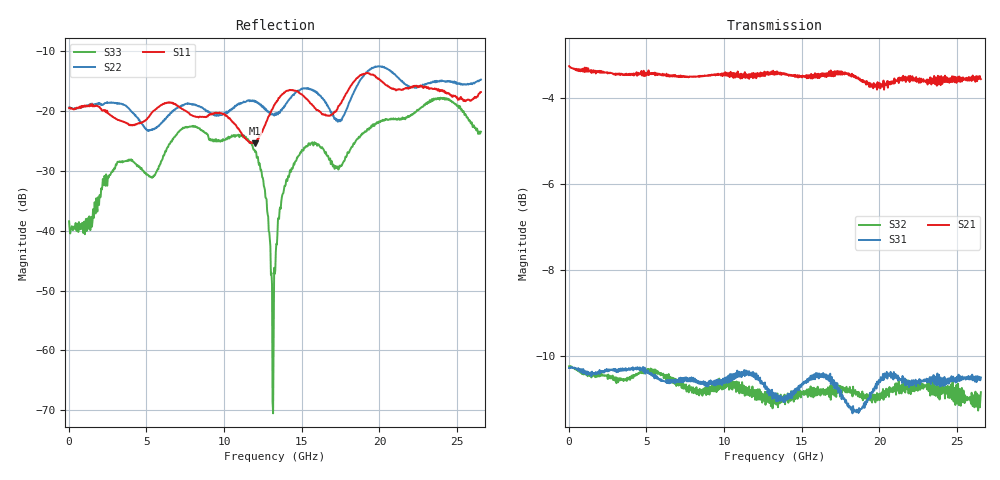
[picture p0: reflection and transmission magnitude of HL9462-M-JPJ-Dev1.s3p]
! 3/13/2020 9:24:54 AM
! H:\PRODUCTION_DATA\TEMP_S3P.S3P
! CHANNEL.1
! TR.MEASUREMENT
! CORRECTED.DATA
# GHZ S RI R 50.0
! FREQ.GHZ  S11RE  S11IM  S12RE  S12IM  S13RE  S13IM
!  S21RE  S21IM  S22RE  S22IM  S23RE  S23IM
!  S31RE  S31IM  S32RE  S32IM  S33RE  S33IM
!; PortSelection: Port_123
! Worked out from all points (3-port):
!   758 points, 35 MHz to 26.53 GHz, reference 50 ohm
!   strongest paths, dB at 35 MHz, 6.65 GHz, 13.3 GHz, 19.91 GHz, 26.53 GHz:
!     S21: -3.3, -3.5, -3.4, -3.7, -3.6
!     S31: -10.3, -10.6, -11.0, -10.7, -10.5
!     S32: -10.2, -10.5, -10.9, -10.9, -10.8
!   lowest |S11| = -25.4 dB at 11.97 GHz (marker M1), VSWR 1.11, Z = 45.1 - j1.28 ohm
!   |S11| at or under -10 dB: start of sweep to end of sweep
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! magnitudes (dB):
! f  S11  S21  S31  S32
! 35 MHz  -19.5  -3.3  -10.3  -10.2
! 7.455 GHz  -19.9  -3.5  -10.5  -10.7
! 11.97 GHz  -25.4  -3.5  -10.4  -10.8
! 12.74 GHz  -21.8  -3.5  -10.7  -10.8
! 13.09 GHz  -19.8  -3.4  -10.8  -10.9
! 13.3 GHz  -18.7  -3.4  -11.0  -10.9
! 13.82 GHz  -17.1  -3.5  -11.1  -11.1
! 15.37 GHz  -18.1  -3.5  -10.5  -10.8
! 23.84 GHz  -16.5  -3.6  -10.4  -10.6
! 26.53 GHz  -16.9  -3.6  -10.5  -10.8
